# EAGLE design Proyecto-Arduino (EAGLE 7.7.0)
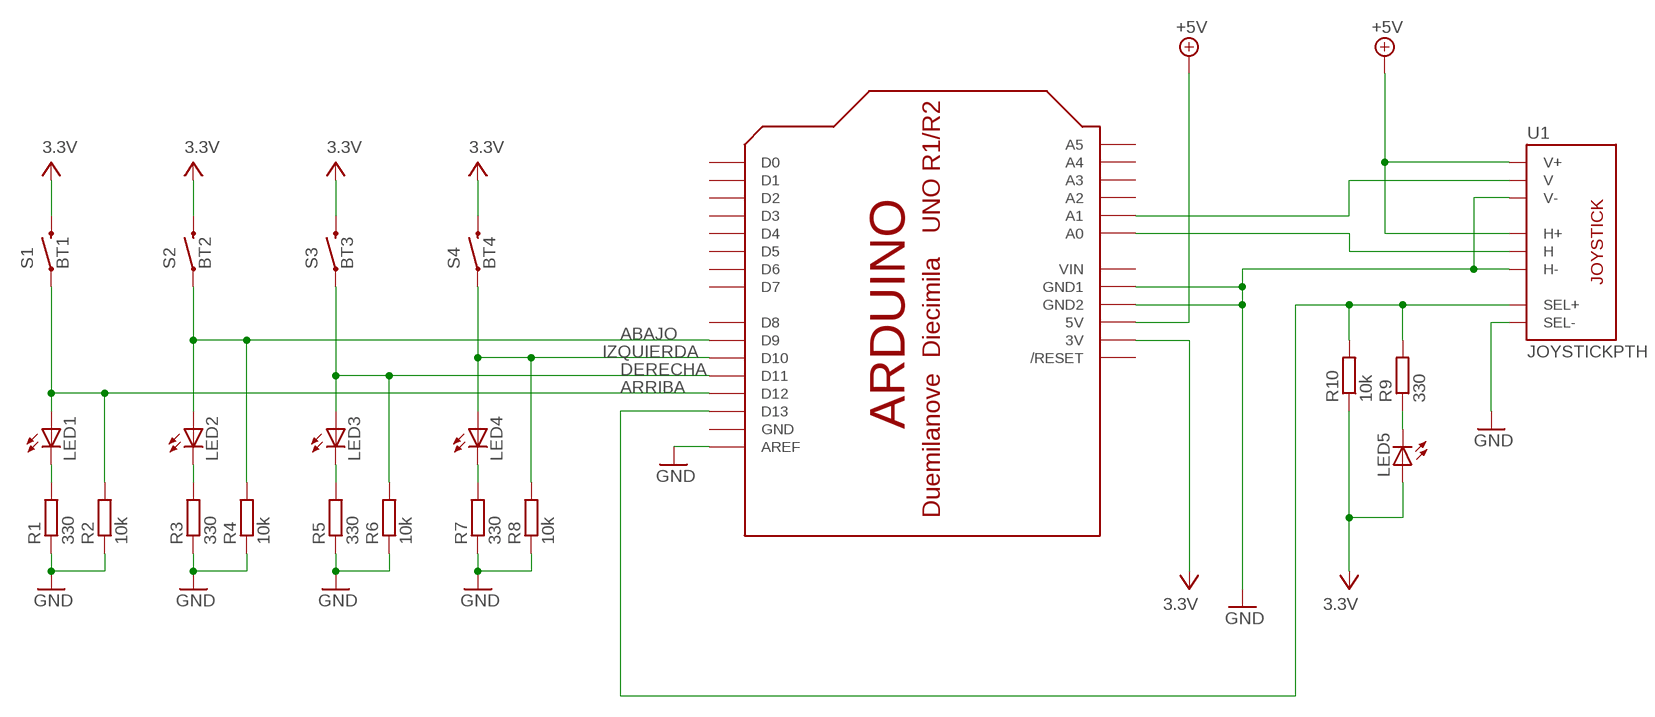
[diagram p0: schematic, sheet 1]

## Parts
LED1  LED3MM  [LED3MM]
LED2  LED3MM  [LED3MM]
LED3  LED3MM  [LED3MM]
LED4  LED3MM  [LED3MM]
LED5  LED3MM  [LED3MM]
R1  330  R  [R0805]
R2  10k  R  [R0805]
R3  330  R  [R0805]
R4  10k  R  [R0805]
R5  330  R  [R0805]
R6  10k  R  [R0805]
R7  330  R  [R0805]
R8  10k  R  [R0805]
R9  330  R  [R0805]
R10  10k  R  [R0805]
S1  BT1  SWITCH-MOMENTARY-212MM  [TACTILE-PTH-12MM]
S2  BT2  SWITCH-MOMENTARY-212MM  [TACTILE-PTH-12MM]
S3  BT3  SWITCH-MOMENTARY-212MM  [TACTILE-PTH-12MM]
S4  BT4  SWITCH-MOMENTARY-212MM  [TACTILE-PTH-12MM]
U1  JOYSTICKPTH  [JOYSTICK]
U$1  ARDUINO-BPLACE  [ARDUINO-BPLACE]

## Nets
+5V: U1.H1(H+) U1.V1(V+) U$1.5V
ABAJO: LED2.A R4.2 S2.1 U$1.D9
ARRIBA: LED1.A R2.2 S1.1 U$1.D12
DERECHA: LED3.A R6.2 S3.1 U$1.D11
GND: R1.1 R2.1 R3.1 R4.1 R5.1 R6.1 R7.1 R8.1 U1.B2A(SEL-) U1.H3(H-) U1.V3(V-) U$1.AREF U$1.GND1 U$1.GND2
IZQUIERDA: LED4.A R8.2 S4.1 U$1.D10
N$1: R9.2 R10.2 U1.B1A(SEL+) U$1.D13
N$2: LED1.K(C) R1.2
N$3: LED5.K(C) R9.1
N$4: LED2.K(C) R3.2
N$5: U1.V2(V) U$1.A1
N$6: LED3.K(C) R5.2
N$7: U1.H2(H) U$1.A0
N$8: LED4.K(C) R7.2
V+: LED5.A R10.1 S1.3 S2.3 S3.3 S4.3 U$1.3V ; supply symbol labelled 3.3V
Unconnected: U$1.A2 U$1.A3 U$1.A4 U$1.A5 U$1.D0 U$1.D1 U$1.D2 U$1.D3 U$1.D4 U$1.D5 U$1.D6 U$1.D7 U$1.D8 U$1.RESET(/RESET)

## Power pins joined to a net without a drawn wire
GND: U$1.GND
VIN: U$1.VIN

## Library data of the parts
LED1-LED5 = adafruit:LED: LED
R1-R10 = eagle-ltspice:R: RESISTOR, European symbol; SPICEMODEL: NONE; SPICEPREFIX: R
S1-S4 = SparkFun-Electromechanical:SWITCH-MOMENTARY-2: Various NO switches- pushbuttons, reed, etc; PROD_ID: SWCH-09185
U1 = adafruit:JOYSTICK: Thumb Joystick Joystick commonly found in PS2 controllers. Two pots and a select switch. Adapted from Sparkfun Library (but for more common 6mm switch sticks)
U$1 = adafruit:ARDUINO: Arduino Diecimila/Duemilanove Make a shield with ease, this package has all the named pins as well as the two mounting drill holes and an outline of the USB and DC power connector. The outline is on the DIMENSION layer, so if your board house uses it they will cut the outline to match.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

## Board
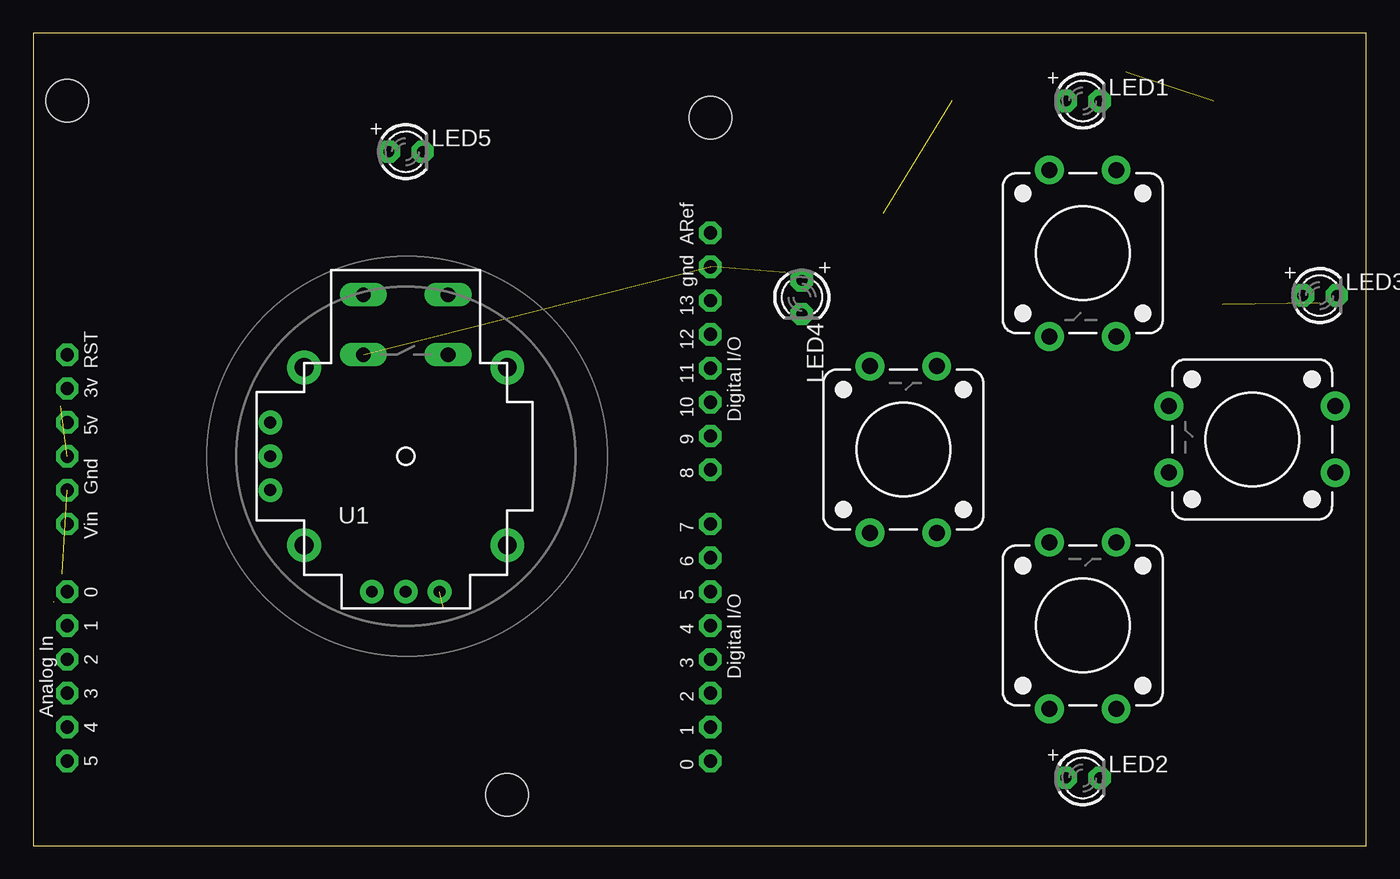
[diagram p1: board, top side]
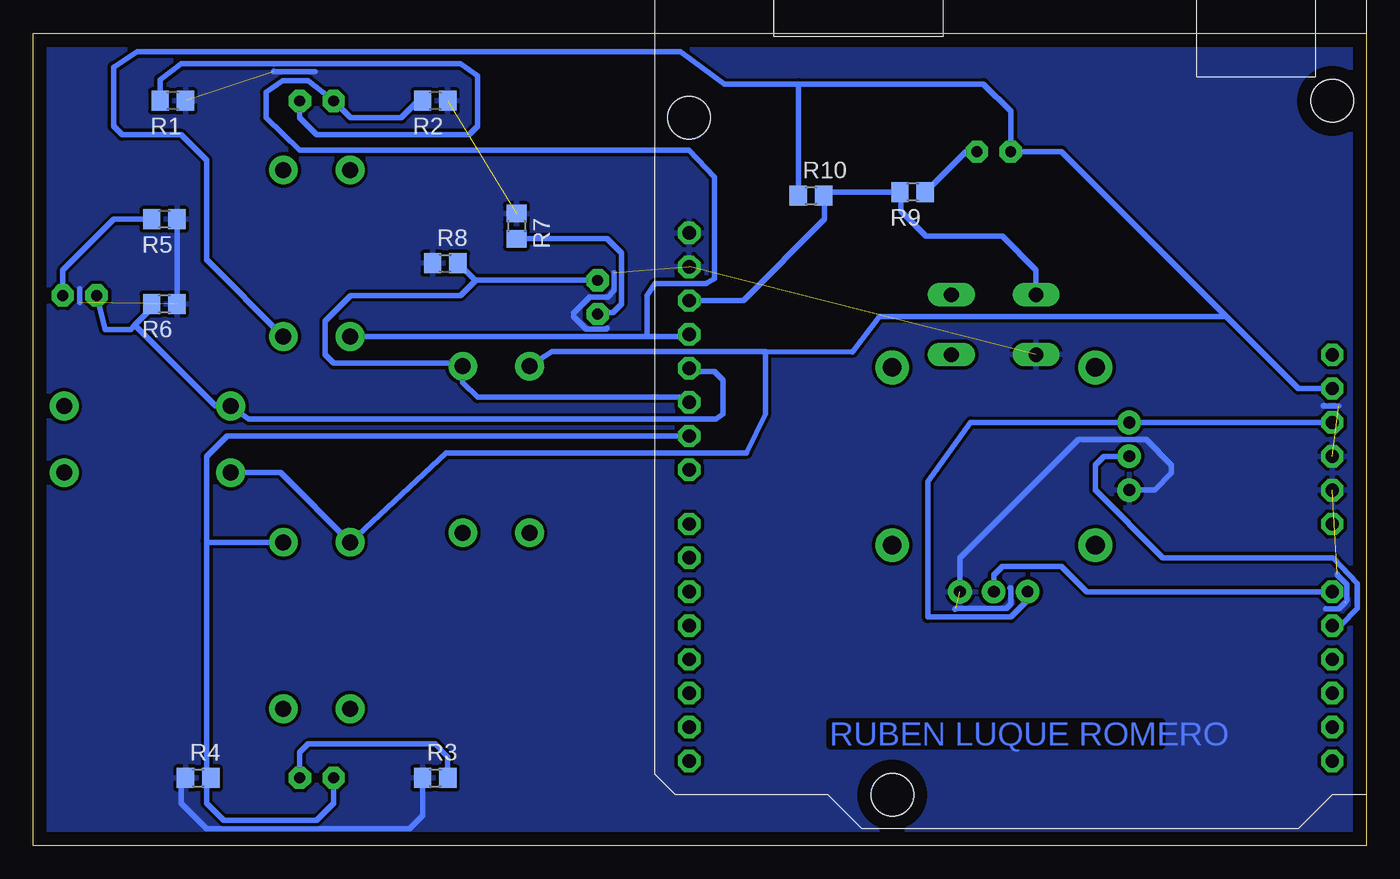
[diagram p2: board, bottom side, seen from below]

Size 100 x 60.95 mm. Coordinates in mm from the lower left corner, seen from the top.
Outline: 0,0 100,0 100,60.95 0,60.95 0,0
Copper layers (1*16): Top 0.035mm / dielectric 1.5mm / Bottom 0.035mm
Design rules "default": minimum track width 10mil, minimum drill 24mil, track to track 8mil, track to pad 8mil, pad to pad 8mil, via to via 8mil, smd to smd 8mil, copper to edge 40mil, drill to drill 8mil, minimum pad ring 10mil, minimum via ring 8mil, stop-mask expansion 4mil, vias tented up to drill 0mil, thermal gap 10mil

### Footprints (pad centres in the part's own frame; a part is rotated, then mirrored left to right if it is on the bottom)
LED3MM = drill 0.813 pad 1.676 octagon: A -1.27,0; K 1.27,0
R0805 = smd 1.3 x 1.5: 1 -0.95,0; 2 0.95,0
TACTILE-PTH-12MM = drill 1.2 pad 2.159: 1 6.25,-2.5; 2 -6.25,-2.5; 3 6.25,2.5; 4 -6.25,2.5
JOYSTICK = drill 1.1 pad 1.778 long: B1A -3.175,12.12; B1B 3.175,12.12; B2A -3.175,7.62; B2B 3.175,7.62 | drill 0.889 pad 1.778: H1 -2.54,-10.16; H2 0,-10.16; H3 2.54,-10.16; V1 -10.16,2.54; V2 -10.16,0; V3 -10.16,-2.54 | drill 1.397 pad 2.54: MOUNT1 -7.62,6.668; MOUNT2 -7.62,-6.668; MOUNT3 7.62,-6.668; MOUNT4 7.62,6.668
ARDUINO-BPLACE = drill 1 pad 1.676 octagon: 3V 35.56,2.54; 5V 38.1,2.54; A0 50.8,2.54; A1 53.34,2.54; A2 55.88,2.54; A3 58.42,2.54; A4 60.96,2.54; A5 63.5,2.54; AREF 23.876,50.8; D0 63.5,50.8; D1 60.96,50.8; D2 58.42,50.8; D3 55.88,50.8; D4 53.34,50.8; D5 50.8,50.8; D6 48.26,50.8; D7 45.72,50.8; D8 41.656,50.8; D9 39.116,50.8; D10 36.576,50.8; D11 34.036,50.8; D12 31.496,50.8; D13 28.956,50.8; GND 26.416,50.8; GND1 43.18,2.54; GND2 40.64,2.54; RESET 33.02,2.54; VIN 45.72,2.54 | hole 3.2: 15.24,50.8; 66.04,35.56; 13.97,2.54

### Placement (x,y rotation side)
LED1  78.74,55.88 0 top
LED2  78.74,5.08 0 top
LED3  96.52,41.27 0 top
LED4  57.66,41.15 270 top
LED5  27.94,52.07 0 top
R1  89.53,55.88 180 bottom
R2  69.85,55.88 180 bottom
R3  69.85,5.08 0 bottom
R4  87.63,5.08 0 bottom
R5  90.17,46.99 180 bottom
R6  90.17,40.64 180 bottom
R7  63.75,46.48 270 bottom
R8  69.09,43.69 0 bottom
R9  34.04,49.02 180 bottom
R10  41.66,48.77 0 bottom
S1  78.74,44.45 270 top
S2  78.74,16.51 90 top
S3  91.44,30.48 180 top
S4  65.28,29.72 90 top
U1  27.94,29.21 0 top
U$1  0,69.85 270 top

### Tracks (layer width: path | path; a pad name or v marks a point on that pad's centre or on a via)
+5V
  Bottom 0.406: U$1.5V U1.V1 29.69,31.75 32.89,27.3 32.89,17.14 26.67,17.14 25.4,18.41 U1.H1
ABAJO
  Bottom 0.406: LED2.A 77.47,3.17 78.74,1.91 85.72,1.91 87,3.17 87,4.76 R4.2 87,5.39 87,22.86 | U$1.D9 85.47,30.73 87,29.21 87,22.86 | S2.1 86.89,22.76 87,22.86
ARRIBA
  Bottom 0.406: R2.2 71.12,55.88 72.39,54.61 76.2,54.61 LED1.A 79.38,57.4 81.28,57.4 82.55,56.52 82.55,54.61 80.01,52.2 50.8,52.2 48.9,50.16 48.9,42.55 49.53,42.16 53.34,42.16 53.98,41.27 53.98,38.2 | S1.1 53.98,38.2 | 53.98,38.2 50.95,38.2 U$1.D12
DERECHA
  Bottom 0.406: R6.2 91.12,40.33 92.39,39.05 | 92.39,39.05 92.71,38.73 94.61,38.73 LED3.A | U$1.D11 50.55,35.56 48.9,35.56 48.26,34.92 48.26,32.38 48.77,32 83.83,32 S3.1 86.32,32.98 92.39,39.05
GND  (9 unrouted)
  Bottom 0.406: R3.1 70.8,2.23 71.75,1.27 87,1.27 88.9,3.17 88.9,4.76 R4.1 | R5.1 R6.1 | U1.H3 30.48,21.59 21.59,30.48 16.51,30.48 14.61,28.57 14.61,27.94 15.88,26.67 U1.V3 | 78.84,58.06 81.97,58.06 81.97,58.12 | 26.75,19.33 26.64,19.33 26.64,18.14 26.67,18.14 27,17.8 30.79,17.8 30.86,17.73 | 56.44,43 56.44,41.63 56.9,41.17 58.27,41.17 59.49,39.95 59.49,39.7 58.55,38.76 57.02,38.76 56.95,38.84 | 2.18,20.37 2.18,20.32 1.45,19.58 1.45,18.39 1.55,18.29 | 2.06,32.97 3.2,32.97 3.2,33.02 | 96.52,41.81 96.52,40.74 | 3.05,17.75 2.06,17.75 1.57,18.24
  pour Bottom (isolate 0.254): 0,60.96 100.33,60.96 100.33,0 0,0
IZQUIERDA
  Bottom 0.406: LED4.A 66.87,42.42 | 66.87,42.42 R8.2 | U$1.D10 51.18,33.66 66.67,33.66 67.78,34.76 S4.1 68,36.2 77.47,36.2 78.11,36.83 78.11,39.37 76.2,41.27 67.94,41.27 66.87,42.35 66.87,42.42
N$1
  Bottom 0.406: U1.B1A 24.77,43.18 27.3,45.72 33.02,45.72 34.92,47.62 34.92,48.96 R9.2 40.45,49.02 R10.2 40.64,48.7 40.64,46.99 46.74,40.89 U$1.D13
N$2
  Bottom 0.406: R1.2 90.48,57.47 88.9,58.67 67.94,58.67 66.67,57.78 66.67,53.98 67.31,53.34 78.74,53.34 80.01,54.61 LED1.K
N$3
  Bottom 0.406: LED5.K 30.04,52.07 R9.1
N$4
  Bottom 0.406: R3.2 68.9,6.67 69.85,7.62 79.38,7.62 80.01,6.99 LED2.K
N$5
  Bottom 0.406: U$1.A1 1.91,16.51 0.69,17.78 0.69,19.68 2.46,21.59 15.24,21.59 20.32,26.67 20.32,28.57 19.68,29.21 U1.V2
N$6
  Bottom 0.406: LED3.K 97.79,43.18 93.98,46.99 R5.2
N$7
  Bottom 0.406: U$1.A0 20.95,19.05 22.86,20.95 27.3,20.95 27.94,20.32 U1.H2
N$8
  Bottom 0.406: R7.2 56.96,45.53 55.88,44.45 55.88,40.64 56.52,40.01 57.53,40.01 LED4.K
V+
  Bottom 0.406: U$1.3V 5.08,34.29 10.48,39.69 | 10.48,39.69 22.86,52.07 LED5.A 26.67,55.12 28.7,57.15 42.55,57.15 | S4.3 61.08,37.08 45.09,37.08 | 45.09,37.08 38.53,37.03 36.51,39.69 10.48,39.69 | 45.09,37.08 45.09,32.38 46.48,29.46 69.03,29.46 S2.3 81.46,27.98 S3.3 | S1.3 87,43.95 87,51.44 88.9,53.34 93.34,53.34 93.98,53.98 93.98,58.42 92.2,59.56 51.44,59.56 48.13,57.15 42.55,57.15 | R10.1 42.61,57.09 42.55,57.15

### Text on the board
Bottom: RUBEN LUQUE ROMERO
